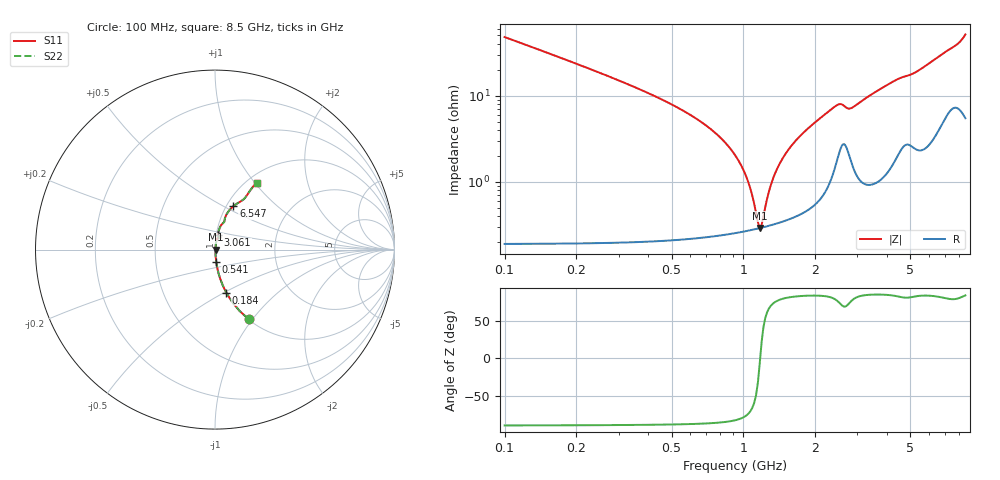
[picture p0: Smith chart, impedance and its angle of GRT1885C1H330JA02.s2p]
!Murata Part Number: GRT1885C1H330JA02
!These Parameters are Measured in Series Mode Connection
!Data Generated on Jun 19, 2026
!  o--ll--o
!Port1  Port2
!  o------o
!Operation Temp=25[degC], DC Bias Voltage=0[V]
!Freq. Start=100[MHz] Stop=9[GHz] 401[Steps]
# Hz S RI R 50
!Freq.(Hz) S11(Real) S11(Imag) S21(Real) S21(Imag) S12(Real) S12(Imag) S22(Real) S22(Imag)
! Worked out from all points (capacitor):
!   401 points, 100 MHz to 8.5 GHz, reference 50 ohm
!   read as one part in series: C = 33 pF near 142 MHz
!   lowest |Z| = 291 mohm at 1.171 GHz (marker M1)
!   series resonance near 1.175 GHz, so ESL is about 560 pH
!   S11 on the Smith chart (normalised r, x): 100 MHz: 1.00, -0.96; 184 MHz: 1.00, -0.51; 541 MHz: 1.00, -0.14; 3.061 GHz: 1.02, +0.16; 6.547 GHz: 1.08, +0.56; 8.5 GHz: 1.11, +1.02
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1e8  0.1875 -0.3883  0.8125 0.3883  0.8125 0.3883  0.1875 -0.3883
1.84e8  0.063 -0.2392  0.937 0.2392  0.937 0.2392  0.063 -0.2392
3.31e8  0.0196 -0.1314  0.9804 0.1314  0.9804 0.1314  0.0196 -0.1314
5.41e8  0.00702 -0.0698  0.993 0.0698  0.993 0.0698  0.00702 -0.0698
7.93e8  0.00346 -0.0331  0.9965 0.0331  0.9965 0.0331  0.00346 -0.0331
9.4e8  0.00289 -0.0185  0.9971 0.0185  0.9971 0.0185  0.00289 -0.0185
1.024e9  0.00279 -0.0114  0.9972 0.0114  0.9972 0.0114  0.00279 -0.0114
1.129e9  0.00283 -0.00331  0.9972 0.00331  0.9972 0.00331  0.00283 -0.00331
1.171e9  0.00289 -0.000295  0.9971 0.000295  0.9971 0.000295  0.00289 -0.000295
1.213e9  0.00296 0.00262  0.997 -0.00262  0.997 -0.00262  0.00296 0.00262
1.339e9  0.0033 0.0109  0.9967 -0.0109  0.9967 -0.0109  0.0033 0.0109
1.507e9  0.00398 0.021  0.996 -0.021  0.996 -0.021  0.00398 0.021
1.822e9  0.00599 0.0386  0.994 -0.0386  0.994 -0.0386  0.00599 0.0386
2.347e9  0.0158 0.0676  0.9842 -0.0676  0.9842 -0.0676  0.0158 0.0676
2.515e9  0.0264 0.0729  0.9736 -0.0729  0.9736 -0.0729  0.0264 0.0729
2.914e9  0.0185 0.0717  0.9815 -0.0717  0.9815 -0.0717  0.0185 0.0717
3.061e9  0.017 0.0802  0.983 -0.0802  0.983 -0.0802  0.017 0.0802
4.3e9  0.0374 0.1402  0.9626 -0.1402  0.9626 -0.1402  0.0374 0.1402
5.707e9  0.0644 0.1961  0.9356 -0.1961  0.9356 -0.1961  0.0644 0.1961
6.547e9  0.1024 0.2416  0.8976 -0.2416  0.8976 -0.2416  0.1024 0.2416
7.114e9  0.137 0.2652  0.863 -0.2652  0.863 -0.2652  0.137 0.2652
8.5e9  0.2315 0.3716  0.7685 -0.3716  0.7685 -0.3716  0.2315 0.3716
